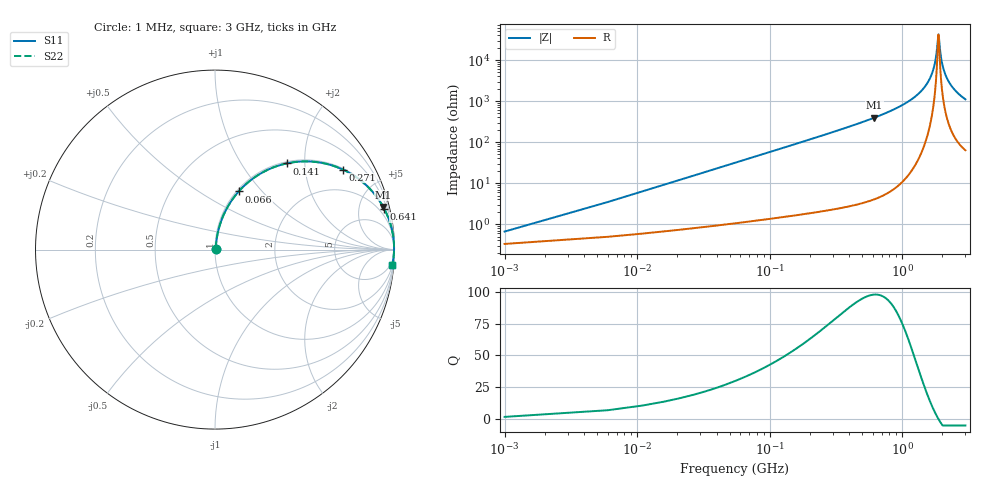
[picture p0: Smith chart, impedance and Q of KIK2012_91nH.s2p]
!version-2
!date-01.2022
!Series
# MHz S RI R 50
!Freq ReS11 ImS11 ReS21 ImS21 ReS12 ImS12 ReS22 ImS22
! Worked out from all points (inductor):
!   601 points, 1 MHz to 3 GHz, reference 50 ohm
!   read as one part in series: L = 91 nH near 16 MHz
!   highest Q = 97.8 at 616 MHz (marker M1), where L = 102 nH
!   self-resonance near 1.876 GHz
!   S11 on the Smith chart (normalised r, x): 1 MHz: 1.01, +0.01; 66 MHz: 1.02, +0.76; 141 MHz: 1.03, +1.62; 271 MHz: 1.04, +3.16; 641 MHz: 1.08, +8.29; 3 GHz: 2, -22
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1  0.00332 0.00568  0.9967 -0.00568  0.9967 -0.00568  0.00332 0.00568
21  0.0212 0.1167  0.9788 -0.1167  0.9788 -0.1167  0.0212 0.1167
26  0.029 0.1433  0.971 -0.1433  0.971 -0.1433  0.029 0.1433
41  0.06 0.2184  0.94 -0.2184  0.94 -0.2184  0.06 0.2184
66  0.1323 0.3242  0.8677 -0.3242  0.8677 -0.3242  0.1323 0.3242
141  0.3986 0.4801  0.6014 -0.4801  0.6014 -0.4801  0.3986 0.4801
271  0.712 0.4461  0.288 -0.4461  0.288 -0.4461  0.712 0.4461
501  0.9024 0.2916  0.0976 -0.2916  0.0976 -0.2916  0.9024 0.2916
616  0.9375 0.237  0.0625 -0.237  0.0625 -0.237  0.9375 0.237
641  0.943 0.2268  0.057 -0.2268  0.057 -0.2268  0.943 0.2268
1001  0.983 0.1228  0.017 -0.1228  0.017 -0.1228  0.983 0.1228
1501  0.9964 0.042  0.0036 -0.042  0.0036 -0.042  0.9964 0.042
1641  0.9974 0.0252  0.00263 -0.0252  0.00263 -0.0252  0.9974 0.0252
1741  0.9977 0.0142  0.00233 -0.0142  0.00233 -0.0142  0.9977 0.0142
1806  0.9977 0.0074  0.00229 -0.0074  0.00229 -0.0074  0.9977 0.0074
1876  0.9977 0.000358  0.00235 -0.000358  0.00235 -0.000358  0.9977 0.000358
1891  0.9976 -0.00112  0.00238 0.00112  0.00238 0.00112  0.9976 -0.00112
1951  0.9975 -0.0069  0.00253 0.0069  0.00253 0.0069  0.9975 -0.0069
2001  0.9973 -0.0116  0.00271 0.0116  0.00271 0.0116  0.9973 -0.0116
2186  0.9963 -0.028  0.00374 0.028  0.00374 0.028  0.9963 -0.028
2501  0.9934 -0.0533  0.00656 0.0533  0.00656 0.0533  0.9934 -0.0533
3000  0.9869 -0.0885  0.0131 0.0885  0.0131 0.0885  0.9869 -0.0885
